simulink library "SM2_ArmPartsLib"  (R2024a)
settings: Solver=ode45  StartTime=0.0  StopTime=10.0  RelTol=1e-3  EnableMultiTasking=on
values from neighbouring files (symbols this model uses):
  m = v*BEAM.rho    [FlexBeamModelConstruct2.m]    (also in FlexBeamModelConstruct3.m = BEAM.rho*v; FlexBeam_1D_Construct.m = REF.m/REF.l*a.*(linspace(1-OPT.MassBiais+1e-6,1+OPT.MassBiai; FlexBeam_3D_Construct.m = REF.m/REF.l*a.*(linspace(1-OPT.MassBiais+1e-6,1+OPT.MassBiai; FreeFlexBeam_3D_Construct.m = REF.m/REF.l*a.*tmp2)
  N = D(1)+(H4^2+H3^2)/H2^2-(E(1)*H4+F(1)*H3)/H2    [MGD.m]    (also in MGD2.m)
  s = -sign(imag(KGZ_fr_tmp))    [LinprogReguliOptimFunc_1.m]    (also in LinprogReguliOptimFunc_2.m; LinprogReguliOptimFunc_1 - Copie.m)
  X = cos(phi(i))*x+sin(phi(i))*y    [MGI.m]
  Y = fft(y(:,i),NFFT)/L    [fft_bis.m]    (also in MGI.m = -sin(phi(i))*x+cos(phi(i))*y)
  Z = z    [MGI.m]
undefined symbols (not defined in the file or in its folder): deg, kg, rad, SimParam
libraries: $bdroot x38, sm_lib x32
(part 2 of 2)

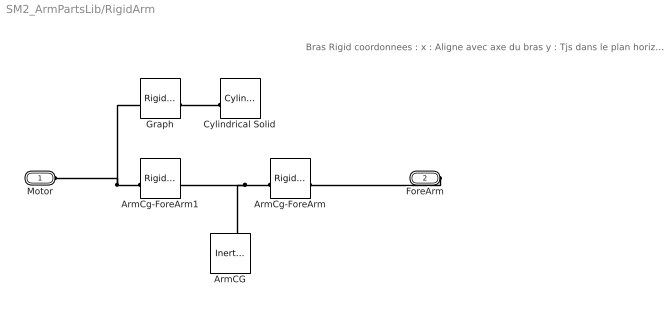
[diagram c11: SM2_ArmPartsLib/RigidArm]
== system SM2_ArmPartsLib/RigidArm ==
  note: Bras Rigid coordonnees : x : Aligne avec axe du bras y : Tjs dans le plan horizontal (Xw,Yw) z : x^y Parametres Solid Longeurs debut-cg : ArmParam.l(1) Longueur cg-fin : ArmParam.l(2) Masse cg : ArmParam.m Inertie cg : ArmParam.I(:)' Rigid transforms Longueur debut-cg : ArmParam.l(1,ID) Longueur cg-fin : ArmParam.l(2,ID)
  ArmCG : sm_lib/Body Elements/Inertia  InertiaType=Custom  Mass=SimParam.Arm.m  MassUnits=kg  CenterOfMass=[0 0 0]  CenterOfMassUnits=m  MomentsOfInertia=SimParam.Arm.I'  MomentsOfInertiaUnits=kg*m^2  ProductsOfInertia=[0 0 0]  ProductsOfInertiaUnits=kg*m^2  GraphicType=Marker  MarkerShape=Inertia  MarkerSize=20  GraphicVisPropType=SimpleVisualProperties  GraphicDiffuseColor=[0.5 0.5 0.5]  GraphicOpacity=1  GraphicSpecularColor=[0.5 0.5 0.5 1.0]  GraphicAmbientColor=[0.15 0.15 0.15 1.0]  GraphicEmissiveColor=[0.0 0.0 0.0 1.0]  GraphicShininess=75
  ArmCg-ForeArm : sm_lib/Frames and Transforms/Rigid Transform  RotationMethod=None  FollAlignAxisA=+X  BaseAlignAxisA=+Y  FollAlignAxisB=+Y  BaseAlignAxisB=+Z  RotationStandardAxis=+Z  RotationAngle=0  RotationAngleUnits=deg  RotationArbitraryAxis=[0 0 1]  RotationSequenceAxes=FollowerAxes  RotationSequence=XYX  RotationSequenceAngles=[0 0 0]  RotationSequenceAnglesUnits=deg  RotationMatrix=[1 0 0;0 1 0;0 0 1]  Quaternion=[1 0 0 0]  TranslationMethod=Cartesian  TranslationCartesianOffset=[SimParam.Arm.l-SimParam.Arm.lcg 0 0]  TranslationCartesianOffsetUnits=m  TranslationStandardAxis=+Z  TranslationStandardOffset=0  TranslationStandardOffsetUnits=m  TranslationROffset=0  TranslationROffsetUnits=m  TranslationThetaOffset=0  TranslationThetaOffsetUnits=deg  TranslationZOffset=0  TranslationZOffsetUnits=m
  ArmCg-ForeArm1 : sm_lib/Frames and Transforms/Rigid Transform  RotationMethod=None  FollAlignAxisA=+X  BaseAlignAxisA=+Y  FollAlignAxisB=+Y  BaseAlignAxisB=+Z  RotationStandardAxis=+Z  RotationAngle=0  RotationAngleUnits=deg  RotationArbitraryAxis=[0 0 1]  RotationSequenceAxes=FollowerAxes  RotationSequence=XYX  RotationSequenceAngles=[0 0 0]  RotationSequenceAnglesUnits=deg  RotationMatrix=[1 0 0;0 1 0;0 0 1]  Quaternion=[1 0 0 0]  TranslationMethod=Cartesian  TranslationCartesianOffset=[SimParam.Arm.lcg 0 0]  TranslationCartesianOffsetUnits=m  TranslationStandardAxis=+Z  TranslationStandardOffset=0  TranslationStandardOffsetUnits=m  TranslationROffset=0  TranslationROffsetUnits=m  TranslationThetaOffset=0  TranslationThetaOffsetUnits=deg  TranslationZOffset=0  TranslationZOffsetUnits=m
  Cylindrical Solid : sm_lib/Body Elements/Cylindrical Solid  CylinderRadius=0.011/2  CylinderRadiusUnits=m  CylinderLength=SimParam.Arm.l  CylinderLengthUnits=m  ExportEntireGeometry=off  InertiaType=CalculateFromGeometry  BasedOnType=Mass  Density=1000  DensityUnits=kg/m^3  Mass=SimParam.Arm.m  MassUnits=kg  CenterOfMass=[0 0 0]  CenterOfMassUnits=m  MomentsOfInertia=[1 1 1]  MomentsOfInertiaUnits=kg*m^2  ProductsOfInertia=[0 0 0]  ProductsOfInertiaUnits=kg*m^2  GraphicType=FromGeometry  MarkerShape=Sphere  MarkerSize=10  GraphicVisPropType=SimpleVisualProperties  GraphicDiffuseColor=[0.5 0.5 0.5]  GraphicOpacity=1  GraphicSpecularColor=[0.5 0.5 0.5 1.0]  GraphicAmbientColor=[0.15 0.15 0.15 1.0]  GraphicEmissiveColor=[0.0 0.0 0.0 1.0]  GraphicShininess=75  DoExposeReferenceFrame=on  SerializedFrames=<Frames/>
  Graph : sm_lib/Frames and Transforms/Rigid Transform  RotationMethod=AlignedAxes  FollAlignAxisA=+Z  BaseAlignAxisA=+X  FollAlignAxisB=+Y  BaseAlignAxisB=+Z  RotationStandardAxis=+Z  RotationAngle=0  RotationAngleUnits=deg  RotationArbitraryAxis=[0 0 1]  RotationSequenceAxes=FollowerAxes  RotationSequence=XYX  RotationSequenceAngles=[0 0 0]  RotationSequenceAnglesUnits=deg  RotationMatrix=[1 0 0;0 1 0;0 0 1]  Quaternion=[1 0 0 0]  TranslationMethod=Cartesian  TranslationCartesianOffset=[SimParam.Arm.l/2 0 0]  TranslationCartesianOffsetUnits=m  TranslationStandardAxis=+Z  TranslationStandardOffset=0  TranslationStandardOffsetUnits=m  TranslationROffset=0  TranslationROffsetUnits=m  TranslationThetaOffset=0  TranslationThetaOffsetUnits=deg  TranslationZOffset=0  TranslationZOffsetUnits=m
  Motor : PMIOPort  Side=Left
  ForeArm : PMIOPort  Port=2  Side=Right
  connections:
  ArmCg-ForeArm/LConn1 -- ArmCG/RConn1 -- ArmCg-ForeArm1/RConn1
  ForeArm/RConn1 -- ArmCg-ForeArm/RConn1
  ArmCg-ForeArm1/LConn1 -- Graph/LConn1 -- Motor/RConn1
  Cylindrical Solid/RConn1 -- Graph/RConn1
